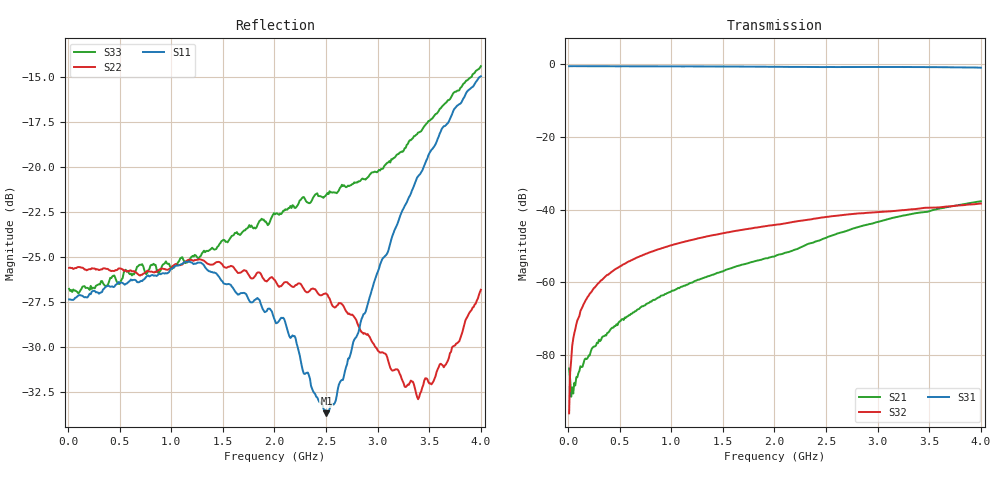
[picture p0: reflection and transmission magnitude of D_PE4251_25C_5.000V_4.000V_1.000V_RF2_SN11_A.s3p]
! Device ID: PE4251_SoldCshunt_081809
! Dir: c:\Test Bench Repositories\Bench_Software_CVI_Version_8\trunk\PSC 4Port_VNA Bench\datalog\4250\TEST\PE4251_SoldCshunt_081809\25C\5p000000\RF2
! Serial: 11
! Insertion: A
! Temp: 25C
! VDD: 5.000
! Control_Hi: 80.000
! Control_Lo: 20.000
! Logic State: RF2
! Port 1: RFC
! Port 2: RF1
! Port 3: RF2
! V1 = 1.00
! V2 = 1.00
! V3 = 1.00
! IDD: 6.323700e-05
! FILE NAME
! DATE 08/18/09  20:14
! CORRECTED  DATA
#  Hz  S  RI  R  50.00
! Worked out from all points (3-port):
!   401 points, 10 MHz to 4 GHz, reference 50 ohm
!   strongest paths, dB at 10 MHz, 1.008 GHz, 2.005 GHz, 3.002 GHz, 4 GHz:
!     S31: -0.5, -0.6, -0.7, -0.8, -1.0
!     S32: -96.1, -49.8, -44.2, -40.7, -38.3
!     S21: -83.7, -62.3, -52.8, -43.4, -37.7
!   lowest |S11| = -33.7 dB at 2.504 GHz (marker M1), VSWR 1.04, Z = 50.5 - j2.01 ohm
!   |S11| at or under -10 dB: start of sweep to end of sweep
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1e7  0.0428 -0.000819  2.77e-05 -3.84e-05  0.9378 -0.00302
     4.79e-05 4.4e-05  0.0524 -0.000838  2.52e-05 -7.35e-05
     0.9389 -0.00429  1.57e-05 6.41e-07  0.0458 0.000356
8.98e7  0.0437 0.00147  2.61e-05 -5.4e-05  0.9387 -0.0321
        1.79e-05 -4.58e-05  0.0526 -0.000967  4.42e-05 0.000288
        0.9394 -0.0324  4.07e-05 0.000295  0.0449 -0.000493
1.696e8  0.0434 0.00224  1.17e-05 -8.24e-05  0.9371 -0.0592
         -1.57e-07 -8.91e-05  0.0519 -0.000761  5.36e-05 0.000565
         0.937 -0.0594  4.54e-05 0.000561  0.0461 0.00143
2.99275e8  0.0443 0.00283  -4.26e-05 -0.000147  0.9323 -0.1046
           -4.44e-05 -0.000155  0.0516 -0.00247  9.27e-05 0.000995
           0.9325 -0.1039  8.38e-05 0.000979  0.0472 -0.000898
4.58875e8  0.0469 0.00171  -0.00015 -0.000208  0.9229 -0.1572
           -0.000137 -0.000208  0.0515 -0.00458  0.000134 0.00149
           0.9243 -0.1581  0.000134 0.00151  0.0487 -0.00541
1.077325e9  0.0521 -0.0116  -0.000773 -0.000331  0.8621 -0.3544
            -0.000761 -0.000321  0.052 -0.0116  0.000508 0.00342
            0.8634 -0.3544  0.000502 0.00342  0.054 -0.00996
2.005e9  0.0349 -0.0134  -0.00224 -0.000435  0.6984 -0.601
         -0.00225 -0.000427  0.0479 -0.00675  0.00114 0.00606
         0.6997 -0.6012  0.00114 0.00606  0.0669 -0.0313
2.50375e9  0.00571 -0.0198  -0.00402 -0.000851  0.5889 -0.6983
           -0.00402 -0.000859  0.0444 0.000588  0.00154 0.00775
           0.5909 -0.6985  0.00155 0.00776  0.0533 -0.0647
3.391525e9  -0.086 -0.0384  -0.00899 0.000935  0.3538 -0.8421
            -0.00897 0.000951  0.0129 0.0185  0.00221 0.01
            0.3546 -0.8413  0.00219 0.01  -0.0254 -0.122
4e9  -0.1767 -0.0269  -0.0126 0.00355  0.1387 -0.8862
     -0.0125 0.00354  -0.0267 0.0369  0.00232 0.0118
     0.1406 -0.8849  0.0023 0.0119  -0.1323 -0.1372
